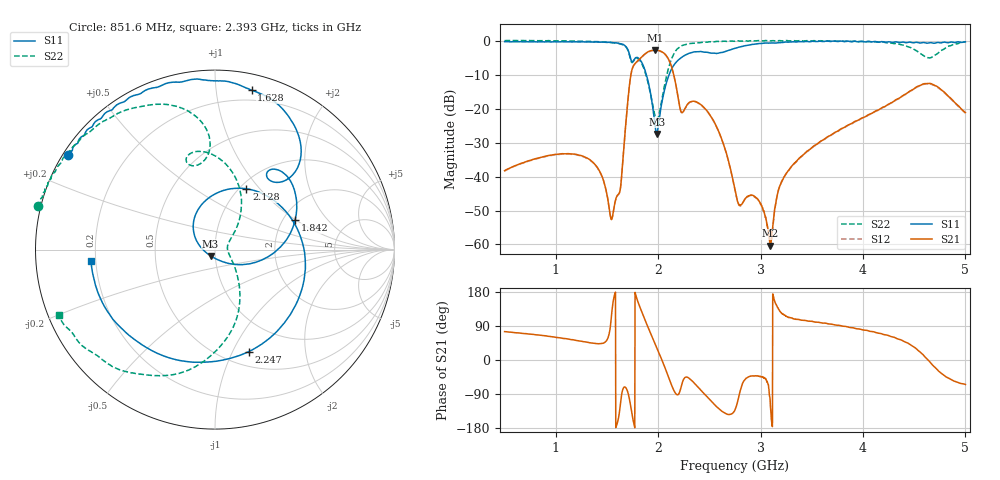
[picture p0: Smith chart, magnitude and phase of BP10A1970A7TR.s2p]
!Agilent Technologies,E8358A,US41080443,A.07.50.56
!Agilent E8358A: A.07.50.56
!Date: Wednesday, July 08, 2015 13:12:09
!Correction: S11(Full 2 Port(1,2))
!S21(Full 2 Port(1,2))
!S12(Full 2 Port(1,2))
!S22(Full 2 Port(1,2))
!S2P File: Measurements: S11, S21, S12, S22:
# Hz S  dB  R 50
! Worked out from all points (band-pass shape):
!   1601 points, 500 MHz to 5 GHz, reference 50 ohm
!   highest |S21| = -2.68 dB at 1.971 GHz (marker M1); lowest = -60.3 dB at 3.093 GHz (marker M2)
!   |S21| within 3 dB of the highest: 1.807 GHz to 2.106 GHz (298.5 MHz wide, 15.3 % of centre)
!   lowest |S11| = -27.4 dB at 1.985 GHz (marker M3), VSWR 1.09, Z = 47.5 - j3.31 ohm
!   |S11| at or under -10 dB: 1.885 GHz to 2.106 GHz (220.8 MHz wide, 11.1 % of centre)
!   |S22| runs from -23.2 to 0.2 dB; largest |S21 - S12| = 0.01
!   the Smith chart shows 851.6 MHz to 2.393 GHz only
!   S11 on the Smith chart (normalised r, x): 851.6 MHz: 0.01, +0.29; 1.628 GHz: 0.12, +1.25; 1.842 GHz: 2.32, +1.00; 2.128 GHz: 1.07, +0.85; 2.247 GHz: 0.65, -1.16; 2.393 GHz: 0.18, -0.04
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5e8  -0.20 161.7  -38.25 75.0  -38.35 75.0  0.10 173.3
8.515625e8  -0.22 147.2  -34.30 65.3  -34.39 65.4  0.11 166.3
1.250938e9  -0.23 124.5  -33.81 49.4  -33.95 49.6  -0.08 153.3
1.540625e9  -0.46 94.2  -52.56 108.9  -52.60 108.5  -0.43 132.6
1.627812e9  -0.81 77.1  -44.04 -123.0  -44.09 -123.1  -0.84 119.3
1.731875e9  -5.41 45.0  -10.21 -122.7  -10.29 -122.7  -5.64 94.7
1.841562e9  -6.43 20.4  -4.60 125.6  -4.73 125.5  -6.81 79.4
1.970938e9  -25.52 -82.7  -2.68 41.4  -2.78 41.4  -22.25 21.2
1.985e9  -27.43 -125.1  -2.71 32.6  -2.80 32.6  -23.14 7.7
2.001875e9  -24.74 -170.4  -2.79 22.1  -2.89 22.0  -22.47 -11.0
2.128438e9  -8.37 62.6  -7.39 -64.9  -7.51 -65.0  -5.45 -86.3
2.246562e9  -4.45 -71.8  -20.74 -51.8  -20.83 -51.9  -1.20 -132.9
2.392812e9  -3.16 -174.8  -18.29 -72.7  -18.38 -72.9  -0.51 -157.2
2.553125e9  -3.61 85.2  -24.23 -118.8  -24.34 -118.3  -0.21 -169.8
2.75e9  -2.17 -22.5  -43.96 -131.7  -44.12 -131.4  -0.07 -179.6
3.093125e9  -0.58 -93.6  -60.34 -106.1  -59.80 -113.9  0.06 169.4
3.500938e9  -0.12 -125.0  -31.43 102.3  -31.54 101.9  0.03 159.4
4.251875e9  -0.24 -166.9  -18.56 64.0  -18.67 63.9  -0.54 126.1
4.485312e9  -0.51 -175.4  -14.33 36.2  -14.46 35.8  -2.25 82.2
4.62875e9  -0.64 -176.7  -12.56 1.8  -12.62 1.8  -4.88 2.4
4.766562e9  -0.53 -178.0  -14.45 -35.4  -14.49 -35.8  -2.76 -92.6
5e9  -0.24 -179.1  -21.11 -64.5  -21.31 -64.5  -0.28 -147.9
